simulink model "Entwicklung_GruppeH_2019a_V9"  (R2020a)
settings: Solver=ode1  StartTime=0.0  StopTime=10.0  FixedStep=0.01  RelTol=1e-3
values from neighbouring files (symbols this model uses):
  Ch = 2.5E5    (= 250000)    [Paramter_Datei_V9.m]
  Cv = 1.2E5    (= 120000)    [Paramter_Datei_V9.m]
  Delta_In = input('Bitte wählen Sie einen Lenkwinkelverlauf aus (1-6): ')    [Paramter_Datei_V9.m]
  Jzz = 3255.86    [Paramter_Datei_V9.m]
  K_delta_v_max = 20    [Paramter_Datei_V9.m]
  l = 2.8    [Paramter_Datei_V9.m]
  LU_ueber = 1    [Paramter_Datei_V9.m]
  lv = 1.45    [Paramter_Datei_V9.m]
  m = 1978    [Paramter_Datei_V9.m]
  V_In = input('Bitte geben Sie eine Geschwindigkeit in km/h ein: ')    [Paramter_Datei_V9.m]
  x = input('Bitte geben Sie den Lenwinkelwert in Grad ein: ')    [Paramter_Datei_V9.m]
libraries: simulink x3, simulink_extras x2

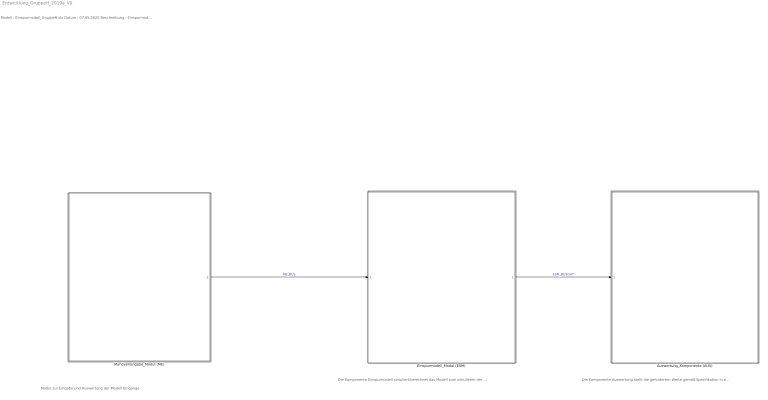
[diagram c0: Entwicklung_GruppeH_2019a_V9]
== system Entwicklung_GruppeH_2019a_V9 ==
  note: Modul zur Eingabe und Auswertung der Modell Eingänge
  note: Die Komponente Auswertung stellt die geforderten Werte gemäß Spezifikation in einem Scope dar
  note: Modell : Einspurmodell_GruppeH.slx Datum : 07.05.2020 Beschreibung : Einspurmodell für die weitere Bearbeitung im Rahmen von Systems Design Engineering (BSE) SS2020 Implementierung : Simulink (R2020a) Toolbox : Standard Simulink Library Autor : Timo Pluls, Lukas Malte Arndt Bemerkung : Modell korriiert nach Komponententest Letzte Änderung : 16.07.2020
  note: Die Komponente Einspurmodell simuliert/berechnet das Modell zum simulieren der Fahrt mit den gegebenen Werten und Patrametern
  Auswertung_Komponente (AUS) : Subsystem
  Einspurmodell_Modul (ESM) : Subsystem
  Manövereingabe_Modul (ME) : Subsystem
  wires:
  Manövereingabe_Modul (ME)/1(ME_BusOut) -> Einspurmodell_Modul (ESM)/1(ME_BUSOUT)  "ME_BUS"
  Einspurmodell_Modul (ESM)/1(ESM_BUSOUT) -> Auswertung_Komponente (AUS)/1(ESM_BUSOUT)  "ESM_BUSOUT"

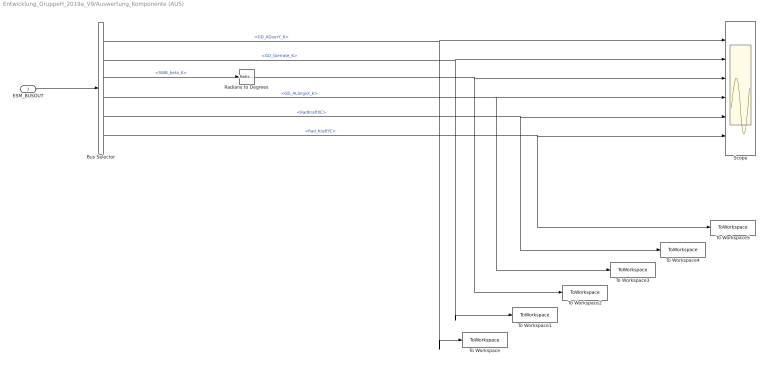
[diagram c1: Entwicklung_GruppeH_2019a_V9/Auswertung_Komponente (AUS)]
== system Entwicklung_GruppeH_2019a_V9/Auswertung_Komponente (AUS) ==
  ESM_BUSOUT : Inport
  Bus Selector : BusSelector  OutputSignals=GD_AQuerY_K,GD_Gierrate_K,SWB_beta_K,GD_ALängsX_K,RadKraftXC,Rad_KraftYC
  Radians to Degrees : simulink_extras/Transformations/Radians to Degrees
  Scope : Scope  NumInputPorts=6
  To Workspace : ToWorkspace  VariableName=AQuer  SaveFormat=Timeseries  SampleTime=-1
  To Workspace1 : ToWorkspace  VariableName=Gierrate  SaveFormat=Timeseries  SampleTime=-1
  To Workspace2 : ToWorkspace  VariableName=beta  SaveFormat=Timeseries  SampleTime=-1
  To Workspace3 : ToWorkspace  VariableName=ALaengs  SaveFormat=Timeseries  SampleTime=-1
  To Workspace4 : ToWorkspace  VariableName=RadKraftXC  SaveFormat=Timeseries  SampleTime=-1
  To Workspace5 : ToWorkspace  VariableName=RadKraftYC  SaveFormat=Timeseries  SampleTime=-1
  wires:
  ESM_BUSOUT/1 -> Bus Selector/1
  Bus Selector/1 -> To Workspace/1, Scope/1  "<GD_AQuerY_K>"
  Bus Selector/2 -> To Workspace1/1, Scope/2  "<GD_Gierrate_K>"
  Bus Selector/3 -> Radians to Degrees/1  "<SWB_beta_K>"
  Bus Selector/4 -> To Workspace3/1, Scope/4  "<GD_ALängsX_K>"
  Bus Selector/5 -> To Workspace4/1, Scope/5  "<RadKraftXC>"
  Bus Selector/6 -> To Workspace5/1, Scope/6  "<Rad_KraftYC>"
  Radians to Degrees/1 -> To Workspace2/1, Scope/3

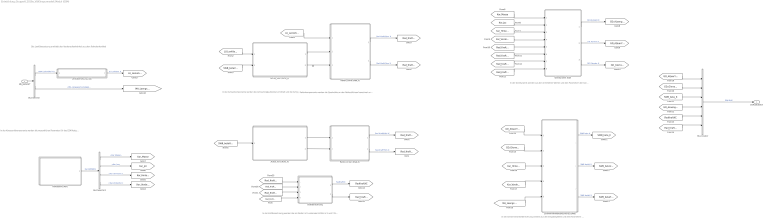
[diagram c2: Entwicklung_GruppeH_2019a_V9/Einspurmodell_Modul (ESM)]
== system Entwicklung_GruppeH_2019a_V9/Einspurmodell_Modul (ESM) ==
  note: In der Kraftberechnung werden die am Reifen in K wirkenden Kräfte in X und Y Richtung in den Schwerpunkt gesetezt
  note: In der Gierdynamik werden aus den ermittelten Werten und den Parametern der Karosserie die aktuelle Gierrate und die Querbeschleunigung berechnet
  note: In der Reifenkomponente werden die Querkräfte an den Reifen/Achsen berechnet und in Bezug zum Koordinantensystem K gesetzt
  note: In der Achsenkomponente werden die Achsschräglaufwinkel ermittelt und die Achsseitensteifigkeiten festfelegt
  note: In der Schwimmwinkelberechnung werden aus den Eingabegrößen und den Parametern des Fahrzeugs der Schwimmwinkel und die Achsschwimmwinkel berechnet
  note: Die Lenkübersetzung ermittelt den Vorderradlenkwinkel aus dem Fahrerlenkwinkel
  note: In der Karosseriekomponente werden die wesentlichen Parameter für das ESM festgelegt
  ME_BUSOUT : Inport
  Achse_hint (Achs_h) : Subsystem
  Achse_vorn (Achs_v) : Subsystem
  Bus Creator : BusCreator  Inputs=6
  Bus Selector : BusSelector  OutputSignals=MA_Lenkwinkel_K,MA_Längsgeschwindigkeit_K
  Bus Selector1 : BusSelector  OutputSignals=Kar_Masse,Kar_Jzz,Kar_HinterZuC,Kar_VorderZuC
  Gierdynamik (GD) : Subsystem
  Karrosserie (Kar) : Subsystem
  Kraftberechnung : Subsystem
  Lenkübersetzung (LU) : Subsystem
  Reifen_hinten (Rad_h) : Subsystem
  Reifen_vorne (Rad_v) : Subsystem
  Schwimmwinkelberechnung (SWB) : Subsystem
  ESM_BUSOUT : Outport
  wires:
  Achse_hint (Achs_h)/1(Achs_SchrägH_K) -> Reifen_hinten (Rad_h)/1(Achs_SchrägH_K)
  Achse_hint (Achs_h)/2(Achs_ChOut) -> Reifen_hinten (Rad_h)/2(Achs_ChOut)
  Achse_vorn (Achs_v)/2(Achs_CvOut) -> Reifen_vorne (Rad_v)/3(Achs_CvOut)
  Bus Creator/1 -> ESM_BUSOUT/1  "ESM_BUS"
  ME_BUSOUT/1 -> Bus Selector/1
  Achse_vorn (Achs_v)/1(Achs_SchrägV_K) -> Reifen_vorne (Rad_v)/2(Achs_SchrägV_K)
  Bus Selector/1 -> Lenkübersetzung (LU)/1(MA_Lenkwinkel)  "<MA_Lenkwinkel_K>"
  Karrosserie (Kar)/1(Kar_DATABUS) -> Bus Selector1/1  "Kar_DATABUS"
  Reifen_hinten (Rad_h)/2(Rad_KraftYHint_K) -> [Rad_KraftYHint_K]  "Rad_KraftYHint_K"
  [Rad_KraftYHint_K] -> Kraftberechnung/4(Rad_KraftYHint_K)
  Reifen_hinten (Rad_h)/1(Rad_KraftXHint_K) -> [Rad_KraftXHint_K]  "Rad_KraftXHint_K"
  [Rad_KraftXHint_K] -> Kraftberechnung/3(Rad_KraftXHint_K)
  Reifen_vorne (Rad_v)/2(Rad_KraftYVorn_K) -> [Rad_KraftYVorn_K]  "Rad_KraftYVorn_K"
  Reifen_vorne (Rad_v)/1(Rad_KraftXVorn_K) -> [Rad_KraftXVorn_K]  "Rad_KraftXVorn_K"
  Bus Selector1/4 -> [Kar_VorderZuC]  "<Kar_VorderZuC>"
  Bus Selector1/3 -> [Kar_HinterZuC]  "<Kar_HinterZuC>"
  Bus Selector1/2 -> [Kar_Jzz]  "<Kar_Jzz>"
  Bus Selector1/1 -> [Kar_Masse]  "<Kar_Masse>"
  Gierdynamik (GD)/1(GD_ALängsX_K) -> [GD_ALaengsX_K]  "GD_ALängsX_K"
  Gierdynamik (GD)/2(GD_AQuerY_K) -> [GD_AQuerY_K]  "GD_AQuerY_K"
  Gierdynamik (GD)/3(GD_Gierrate_K) -> [GD_Gierrate_K]  "GD_Gierrate_K"
  Schwimmwinkelberechnung (SWB)/1(SWB_beta_K) -> [SWB_beta_K]  "SWB_beta_K"
  Schwimmwinkelberechnung (SWB)/2(SWB_betaV_K) -> [SWB_betaV_K]  "SWB_betaV_K"
  Schwimmwinkelberechnung (SWB)/3(SWB_betaH_) -> [SWB_betaH_K]  "SWB_betaH_K"
  Kraftberechnung/1(Rad_KraftXC) -> [RadKraftXC]  "RadKraftXC"
  Kraftberechnung/2(Rad_KraftYC) -> [Rad_KraftYC]
  Bus Selector/2 -> [MA_Laengsgeschwindigkeit_K]  "<MA_Längsgeschwindigkeit_K>"
  Lenkübersetzung (LU)/1(LU_LenkVorn_K) -> [LU_LenkVorn_K]  "LU_LenkVorn_K"
  [LU_LenkVorn_K] -> Achse_vorn (Achs_v)/1(LU_LenkVorn)
  [SWB_betaV_K] -> Achse_vorn (Achs_v)/2(SWB_betV)
  [LU_LenkVorn_K] -> Reifen_vorne (Rad_v)/1(LU_LenkVorn_K)
  [SWB_betaH_K] -> Achse_hint (Achs_h)/1(SWB_betaH)
  [Kar_Masse] -> Gierdynamik (GD)/1(Kar_Masse)
  [Kar_Jzz] -> Gierdynamik (GD)/2(Kar_Jzz)
  [Kar_HinterZuC] -> Gierdynamik (GD)/3("Kar_HinterzuC ")
  [Kar_VorderZuC] -> Gierdynamik (GD)/4(Kar_VorderZuC)
  [Rad_KraftXVorn_K] -> Gierdynamik (GD)/5(Rad_KraftXVorn_K)
  [Rad_KraftYVorn_K] -> Gierdynamik (GD)/6(Rad_KraftYVorn_K)
  [Rad_KraftYHint_K] -> Gierdynamik (GD)/7(Rad_KraftYHint_K)
  [Rad_KraftXHint_K] -> Gierdynamik (GD)/8(Rad_KraftXHint_K)
  [GD_AQuerY_K] -> Schwimmwinkelberechnung (SWB)/1(GD_AQuerY_K)
  [GD_Gierrate_K] -> Schwimmwinkelberechnung (SWB)/2("GD_Gierrate_K ")
  [Kar_HinterZuC] -> Schwimmwinkelberechnung (SWB)/3(<Kar_HinterZuC>)
  [Kar_VorderZuC] -> Schwimmwinkelberechnung (SWB)/4(<Kar_VorderZuC>)
  [MA_Laengsgeschwindigkeit_K] -> Schwimmwinkelberechnung (SWB)/5(<MA_Längsgeschwindigkeit_K>)
  [GD_AQuerY_K] -> Bus Creator/1
  [GD_Gierrate_K] -> Bus Creator/2
  [SWB_beta_K] -> Bus Creator/3
  [GD_ALaengsX_K] -> Bus Creator/4
  [RadKraftXC] -> Bus Creator/5
  [Rad_KraftYC] -> Bus Creator/6
  [Rad_KraftXVorn_K] -> Kraftberechnung/1(Rad_KraftXVorn_K)
  [Rad_KraftYVorn_K] -> Kraftberechnung/2(Rad_KraftYVorn_K)

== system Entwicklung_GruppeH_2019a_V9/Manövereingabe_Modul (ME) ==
  note: In der Komponente Manöverauswahl werden die User_Input_Signale interpretiert und die zugehörigen Werte Geschwindigkeit und Lenkwinkel ermittelt
  Bus Creator : BusCreator  Inputs=2
  Constant : Constant  Value=V_In
  Constant1 : Constant  Value=Delta_In
  Manöverauswahl (MA) : Subsystem
  ME_BusOut : Outport
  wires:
  Constant1/1 -> Manöverauswahl (MA)/1(ME_LenkwinkelIn)
  Constant/1 -> Manöverauswahl (MA)/2(ME_GeschwIn)
  Manöverauswahl (MA)/1(MA_Lenkwinkel_K) -> Bus Creator/1  "MA_Lenkwinkel_K"
  Manöverauswahl (MA)/2(MA_Längsgeschwindigkeit_K) -> Bus Creator/2  "MA_Längsgeschwindigkeit_K"
  Bus Creator/1 -> ME_BusOut/1  "ME_BUS"

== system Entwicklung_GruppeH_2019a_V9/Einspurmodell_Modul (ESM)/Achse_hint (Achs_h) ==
  SWB_betaH : Inport
  Achs_ChPar : Constant  Value=Ch
  Gain : Gain  Gain=-1
  Achs_SchrägH_K : Outport
  Achs_ChOut : Outport  Port=2
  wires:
  Achs_ChPar/1 -> Achs_ChOut/1
  Gain/1 -> Achs_SchrägH_K/1
  SWB_betaH/1 -> Gain/1

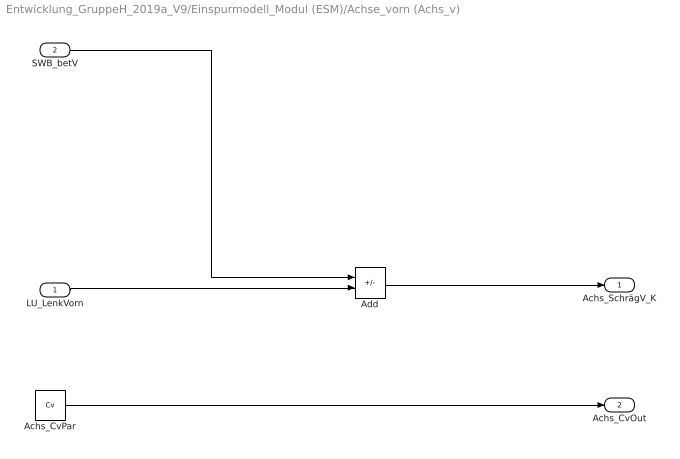
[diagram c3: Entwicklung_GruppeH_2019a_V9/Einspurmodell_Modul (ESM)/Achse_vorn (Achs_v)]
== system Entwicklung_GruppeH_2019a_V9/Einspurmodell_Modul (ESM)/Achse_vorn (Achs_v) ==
  LU_LenkVorn : Inport
  SWB_betV : Inport  Port=2
  Achs_CvPar : Constant  Value=Cv
  Add : Sum  Inputs=-+
  Achs_SchrägV_K : Outport
  Achs_CvOut : Outport  Port=2
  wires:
  Achs_CvPar/1 -> Achs_CvOut/1
  Add/1 -> Achs_SchrägV_K/1
  LU_LenkVorn/1 -> Add/2
  SWB_betV/1 -> Add/1

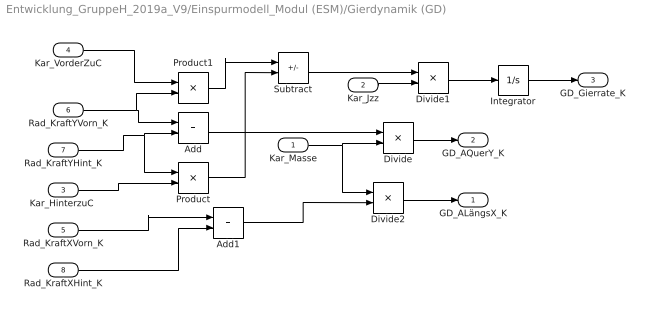
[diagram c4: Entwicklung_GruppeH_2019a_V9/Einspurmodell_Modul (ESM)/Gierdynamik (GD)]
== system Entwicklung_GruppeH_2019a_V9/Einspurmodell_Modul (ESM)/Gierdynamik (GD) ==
  Kar_Masse : Inport
  Kar_Jzz : Inport  Port=2
  "Kar_HinterzuC " : Inport  Port=3
  Kar_VorderZuC : Inport  Port=4
  Rad_KraftXVorn_K : Inport  Port=5
  Rad_KraftYVorn_K : Inport  Port=6
  Rad_KraftYHint_K : Inport  Port=7
  Rad_KraftXHint_K : Inport  Port=8
  Add : Sum
  Add1 : Sum
  Divide : Product  Inputs=*/
  Divide1 : Product  Inputs=*/
  Divide2 : Product  Inputs=/*
  Integrator : Integrator
  Product : Product
  Product1 : Product
  Subtract : Sum  Inputs=+-
  GD_ALängsX_K : Outport
  GD_AQuerY_K : Outport  Port=2
  GD_Gierrate_K : Outport  Port=3
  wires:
  Rad_KraftYVorn_K/1 -> Product1/2, Add/1
  Rad_KraftYHint_K/1 -> Product/1, Add/2
  Add/1 -> Divide/1
  Kar_Masse/1 -> Divide2/1, Divide/2
  Kar_VorderZuC/1 -> Product1/1
  "Kar_HinterzuC "/1 -> Product/2
  Product1/1 -> Subtract/1
  Product/1 -> Subtract/2
  Subtract/1 -> Divide1/1
  Kar_Jzz/1 -> Divide1/2
  Divide1/1 -> Integrator/1
  Integrator/1 -> GD_Gierrate_K/1
  Divide/1 -> GD_AQuerY_K/1
  Rad_KraftXVorn_K/1 -> Add1/1
  Rad_KraftXHint_K/1 -> Add1/2
  Add1/1 -> Divide2/2
  Divide2/1 -> GD_ALängsX_K/1

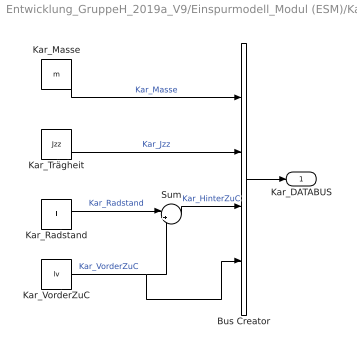
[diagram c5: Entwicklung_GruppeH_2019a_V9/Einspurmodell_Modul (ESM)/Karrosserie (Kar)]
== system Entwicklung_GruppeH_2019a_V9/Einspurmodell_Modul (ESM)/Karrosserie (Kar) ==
  Bus Creator : BusCreator  Inputs=4
  Kar_Masse : Constant  Value=m
  Kar_Radstand : Constant  Value=l
  Kar_Trägheit : Constant  Value=Jzz
  Kar_VorderZuC : Constant  Value=lv
  Sum : Sum  Inputs=|+-
  Kar_DATABUS : Outport
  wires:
  Kar_VorderZuC/1 -> Bus Creator/4, Sum/2  "Kar_VorderZuC"
  Kar_Radstand/1 -> Sum/1  "Kar_Radstand"
  Kar_Trägheit/1 -> Bus Creator/2  "Kar_Jzz"
  Kar_Masse/1 -> Bus Creator/1  "Kar_Masse"
  Bus Creator/1 -> Kar_DATABUS/1
  Sum/1 -> Bus Creator/3  "Kar_HinterZuC"

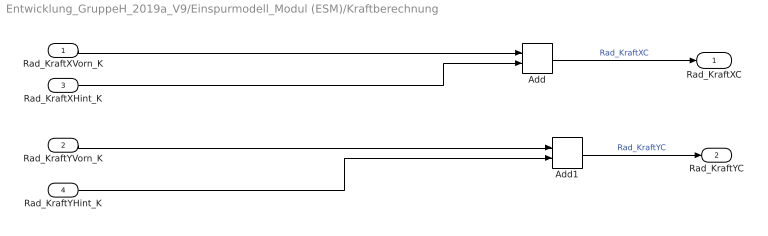
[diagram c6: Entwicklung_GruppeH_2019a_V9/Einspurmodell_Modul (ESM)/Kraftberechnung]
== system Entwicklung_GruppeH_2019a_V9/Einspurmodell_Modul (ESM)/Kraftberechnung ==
  Rad_KraftXVorn_K : Inport
  Rad_KraftYVorn_K : Inport  Port=2
  Rad_KraftXHint_K : Inport  Port=3
  Rad_KraftYHint_K : Inport  Port=4
  Add : Sum
  Add1 : Sum
  Rad_KraftXC : Outport
  Rad_KraftYC : Outport  Port=2
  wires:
  Add/1 -> Rad_KraftXC/1  "Rad_KraftXC"
  Add1/1 -> Rad_KraftYC/1  "Rad_KraftYC"
  Rad_KraftXVorn_K/1 -> Add/1
  Rad_KraftXHint_K/1 -> Add/2
  Rad_KraftYVorn_K/1 -> Add1/1
  Rad_KraftYHint_K/1 -> Add1/2

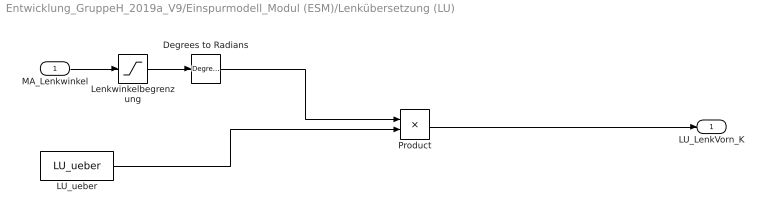
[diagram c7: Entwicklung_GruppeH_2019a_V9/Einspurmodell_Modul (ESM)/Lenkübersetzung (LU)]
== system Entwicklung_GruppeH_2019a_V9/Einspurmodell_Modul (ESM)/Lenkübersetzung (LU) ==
  MA_Lenkwinkel : Inport
  Degrees to Radians : simulink_extras/Transformations/Degrees to Radians
  LU_ueber : Constant  Value=LU_ueber
  Lenkwinkelbegrenzung : Saturate  UpperLimit=K_delta_v_max  LowerLimit=-K_delta_v_max
  Product : Product
  LU_LenkVorn_K : Outport
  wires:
  LU_ueber/1 -> Product/2
  Degrees to Radians/1 -> Product/1
  MA_Lenkwinkel/1 -> Lenkwinkelbegrenzung/1
  Lenkwinkelbegrenzung/1 -> Degrees to Radians/1
  Product/1 -> LU_LenkVorn_K/1

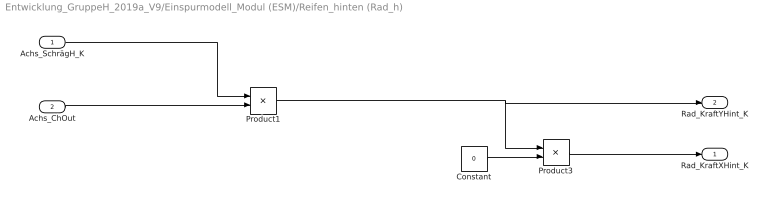
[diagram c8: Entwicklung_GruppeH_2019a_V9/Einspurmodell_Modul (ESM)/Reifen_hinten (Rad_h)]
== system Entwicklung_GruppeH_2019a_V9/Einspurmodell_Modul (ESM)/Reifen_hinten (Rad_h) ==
  Achs_SchrägH_K : Inport
  Achs_ChOut : Inport  Port=2
  Constant : Constant  Value=0
  Product1 : Product
  Product3 : Product
  Rad_KraftXHint_K : Outport
  Rad_KraftYHint_K : Outport  Port=2
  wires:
  Achs_ChOut/1 -> Product1/2
  Achs_SchrägH_K/1 -> Product1/1
  Product1/1 -> Product3/1, Rad_KraftYHint_K/1
  Constant/1 -> Product3/2
  Product3/1 -> Rad_KraftXHint_K/1

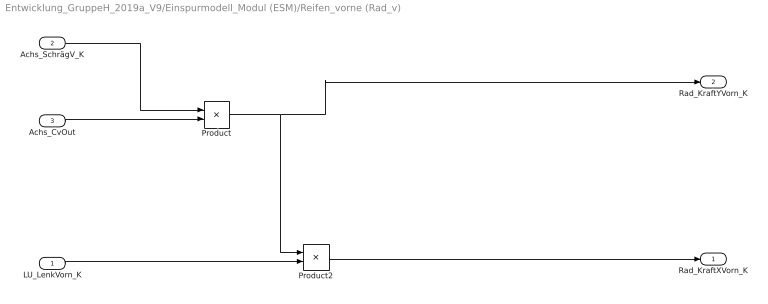
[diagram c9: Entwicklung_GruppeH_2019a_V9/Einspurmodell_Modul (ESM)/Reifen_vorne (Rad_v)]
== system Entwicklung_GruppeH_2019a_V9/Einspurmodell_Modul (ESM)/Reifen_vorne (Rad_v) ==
  LU_LenkVorn_K : Inport
  Achs_SchrägV_K : Inport  Port=2
  Achs_CvOut : Inport  Port=3
  Product : Product
  Product2 : Product
  Rad_KraftXVorn_K : Outport
  Rad_KraftYVorn_K : Outport  Port=2
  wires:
  Achs_CvOut/1 -> Product/2
  Achs_SchrägV_K/1 -> Product/1
  Product/1 -> Product2/1, Rad_KraftYVorn_K/1
  LU_LenkVorn_K/1 -> Product2/2
  Product2/1 -> Rad_KraftXVorn_K/1

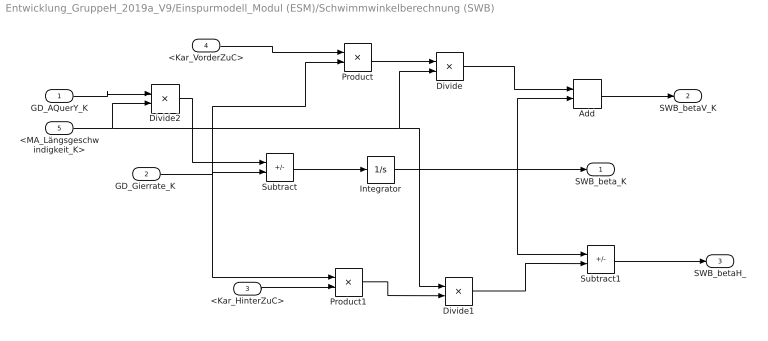
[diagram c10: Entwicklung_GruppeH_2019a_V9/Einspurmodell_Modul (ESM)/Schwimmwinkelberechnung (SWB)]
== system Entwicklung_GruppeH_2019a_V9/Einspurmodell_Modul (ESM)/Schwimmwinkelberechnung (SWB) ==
  GD_AQuerY_K : Inport
  "GD_Gierrate_K " : Inport  Port=2
  <Kar_HinterZuC> : Inport  Port=3
  <Kar_VorderZuC> : Inport  Port=4
  <MA_Längsgeschwindigkeit_K> : Inport  Port=5
  Add : Sum
  Divide : Product  Inputs=*/
  Divide1 : Product  Inputs=/*
  Divide2 : Product  Inputs=*/
  Integrator : Integrator
  Product : Product
  Product1 : Product
  Subtract : Sum  Inputs=+-
  Subtract1 : Sum  Inputs=+-
  SWB_beta_K : Outport
  SWB_betaV_K : Outport  Port=2
  SWB_betaH_ : Outport  Port=3
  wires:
  Integrator/1 -> Add/2, Subtract1/1, SWB_beta_K/1
  "GD_Gierrate_K "/1 -> Product1/1, Product/2, Subtract/2
  Subtract/1 -> Integrator/1
  <Kar_VorderZuC>/1 -> Product/1
  Product/1 -> Divide/1
  <MA_Längsgeschwindigkeit_K>/1 -> Divide2/2, Divide1/1, Divide/2
  Divide/1 -> Add/1
  Add/1 -> SWB_betaV_K/1
  Subtract1/1 -> SWB_betaH_/1
  <Kar_HinterZuC>/1 -> Product1/2
  Product1/1 -> Divide1/2
  Divide1/1 -> Subtract1/2
  GD_AQuerY_K/1 -> Divide2/1
  Divide2/1 -> Subtract/1

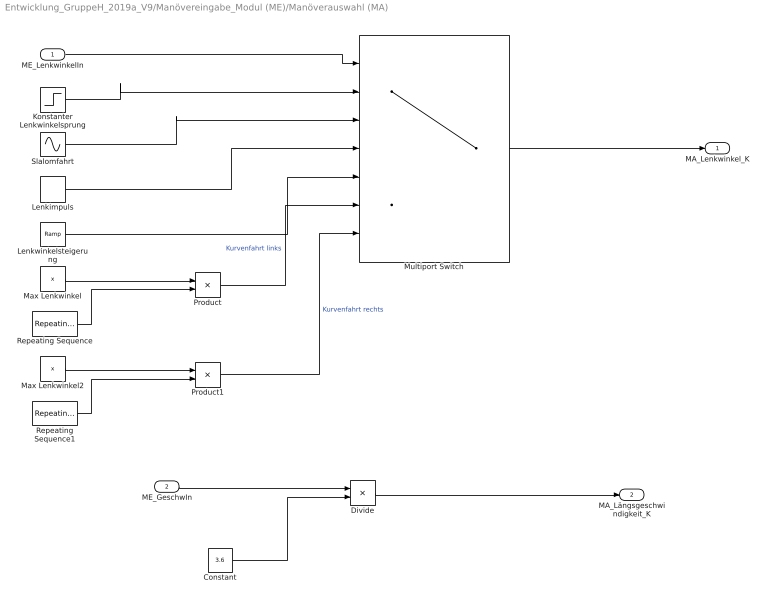
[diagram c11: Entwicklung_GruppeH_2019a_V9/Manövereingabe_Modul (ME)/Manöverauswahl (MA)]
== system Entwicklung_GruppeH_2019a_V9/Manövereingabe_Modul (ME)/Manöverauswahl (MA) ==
  ME_LenkwinkelIn : Inport
  ME_GeschwIn : Inport  Port=2
  Constant : Constant  Value=3.6
  Divide : Product  Inputs=*/
  Konstanter Lenkwinkelsprung : Step  After=x  SampleTime=0
  Lenkimpuls : DiscretePulseGenerator  PulseType=Time based  Amplitude=x  Period=10  PulseWidth=5
  Lenkwinkelsteigerung : simulink/Sources/Ramp  slope=1  start=0  InitialOutput=0
  Max Lenkwinkel : Constant  Value=x
  Max Lenkwinkel2 : Constant  Value=x
  Multiport Switch : MultiPortSwitch  Inputs=6
  Product : Product
  Product1 : Product
  Repeating Sequence : simulink/Sources/Repeating Sequence  rep_seq_t=t  rep_seq_y=Kurve_Links
  Repeating Sequence1 : simulink/Sources/Repeating Sequence  rep_seq_t=t  rep_seq_y=Kurve_Rechts
  Slalomfahrt : Sin  Amplitude=x  SampleTime=0
  MA_Lenkwinkel_K : Outport
  MA_Längsgeschwindigkeit_K : Outport  Port=2
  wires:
  ME_GeschwIn/1 -> Divide/1
  Constant/1 -> Divide/2
  Divide/1 -> MA_Längsgeschwindigkeit_K/1
  ME_LenkwinkelIn/1 -> Multiport Switch/1
  Konstanter Lenkwinkelsprung/1 -> Multiport Switch/2
  Slalomfahrt/1 -> Multiport Switch/3
  Lenkimpuls/1 -> Multiport Switch/4
  Lenkwinkelsteigerung/1 -> Multiport Switch/5
  Max Lenkwinkel/1 -> Product/1
  Repeating Sequence/1 -> Product/2
  Product/1 -> Multiport Switch/6  "Kurvenfahrt links"
  Max Lenkwinkel2/1 -> Product1/1
  Product1/1 -> Multiport Switch/7  "Kurvenfahrt rechts"
  Repeating Sequence1/1 -> Product1/2
  Multiport Switch/1 -> MA_Lenkwinkel_K/1
